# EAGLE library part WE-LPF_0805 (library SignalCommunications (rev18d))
Multilayer Chip Low-Pass Filter Characteristics Operating temperature: –40 °C to +85 °C Power capacity up to 3 W Low insertion loss and high attenuation in the stop-band Applications RF applications Wireless communication systems like DECT, PACS, PHS, GSM, WLAN, Bluetooth … Details see: http://katalog.we-online.de/en/pbs/WE-LPF? Updated by Dan Xu 2014-07-08 2014 (C) Wurth Elektronik
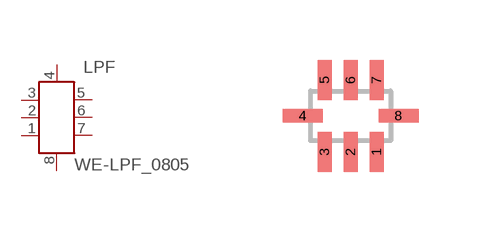
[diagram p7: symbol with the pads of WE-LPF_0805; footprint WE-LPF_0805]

Designator prefix LPF

## WE-LPF_0805_748111009, WE-LPF_0805_748121055, WE-LPF_0805_748125024  [WE-LPF_0805]
1  GND1  pwr
2  NC  nc
3  GND2  pwr
4  OUT  out
5  GND3  pwr
6  NC1  nc
7  GND4  pwr
8  IN  in

## Footprint WE-LPF_0805 (pad centres in mm)
Multilayer Chip Low-Pass Filters WE-LPF
smd 0.35 x 1: 1 0.65,-0.9; 2 0,-0.9; 3 -0.65,-0.9; 5 -0.65,0.9; 6 0,0.9; 7 0.65,0.9
smd 1 x 0.35: 4 -1.2,0; 8 1.2,0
